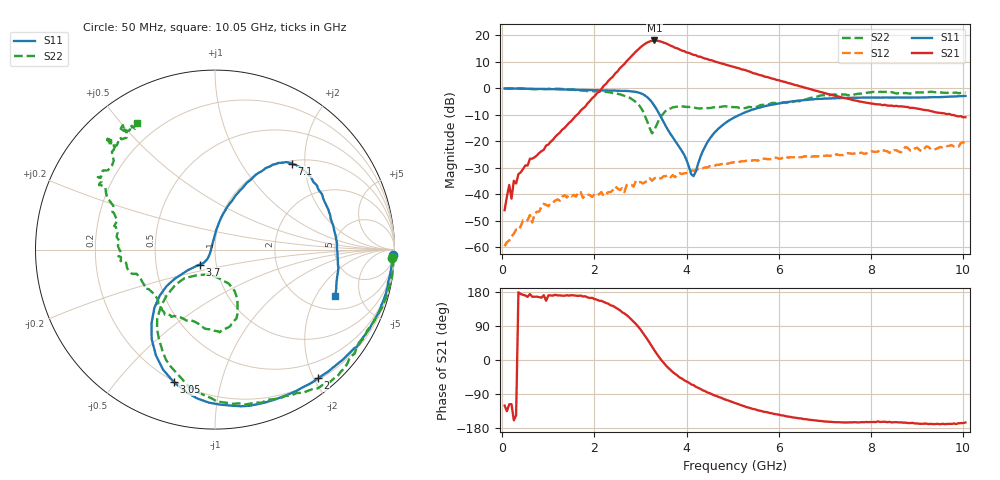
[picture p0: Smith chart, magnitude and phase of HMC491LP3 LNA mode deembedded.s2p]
!Hittite Microwave Corporation
!12 Elizabeth Drive
!Chelmsford, MA 01824
!Tel: 978-250-3343
!Fax: 978-250-3373
!Device: HMC491LP3, 3.4-3.8 GHz, GaAs MMIC Low Noise Amplifier with Bypass Mode in leadless SMT package
!Misc: LNA Mode, Room
# MHZ S MA R 50
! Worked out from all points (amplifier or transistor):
!   201 points, 50 MHz to 10.05 GHz, reference 50 ohm
!   highest |S21| = 18.0 dB at 3.3 GHz (marker M1)
!   |S21| within 3 dB of that: 2.973 GHz to 3.802 GHz (828.6 MHz wide, 24.5 % of centre)
!   unconditionally stable (mu >= 1): start of sweep to 1.123 GHz; 1.331 GHz to 2.286 GHz; 2.979 GHz to end of sweep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
!   at 1.7 GHz: K = 2.02, MAG = 9.6 dB, |S12| = -39.2 dB
!   at 5.05 GHz: K = 3.87, MAG = 9.1 dB, |S12| = -28.0 dB
!   at 10.05 GHz: K = 2.52, MAG = -1.8 dB, |S12| = -21.0 dB
!   S11 on the Smith chart (normalised r, x): 50 MHz: 17, -58; 2 GHz: 0.23, -2.06; 3.05 GHz: 0.20, -0.72; 3.7 GHz: 0.83, -0.14; 7.1 GHz: 1.06, +1.73; 10.05 GHz: 2.74, -2.93
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50  0.991 -1.8  0.005002 -120.3  0.00105 -2.1  0.99 -2.7
150  0.989 -4.2  0.015 -116.9  0.001341 61.9  0.995 -6.6
1750  0.929 -45.3  0.415 167.5  0.008565 88.3  0.904 -66.7
2000  0.918 -51.3  0.707 160.7  0.009968 73.9  0.88 -77.3
2400  0.904 -63.6  1.66 142.9  0.012 80.8  0.814 -94.1
2700  0.891 -77.5  3.256 118.4  0.015 68.5  0.695 -111.0
2900  0.853 -92.3  4.928 94.9  0.018 46.8  0.549 -126.1
3050  0.772 -107.4  6.445 71.7  0.016 22.1  0.372 -136.5
3150  0.674 -119.3  7.335 54.3  0.018 5.9  0.232 -136.8
3300  0.469 -136.1  7.988 25.8  0.02 -26.2  0.163 -81.3
3400  0.337 -143.0  7.763 8.0  0.02 -53.4  0.255 -64.7
3550  0.192 -142.9  7.056 -14.2  0.022 -76.7  0.378 -70.6
3700  0.119 -135.4  6.144 -32.0  0.023 -95.5  0.436 -78.9
3950  0.055 -131.6  5.011 -53.7  0.025 -115.7  0.452 -90.4
4150  0.022 160.0  4.272 -66.3  0.028 -127.6  0.437 -98.9
4350  0.065 94.8  3.767 -80.1  0.031 -133.7  0.423 -110.7
5050  0.287 70.8  2.496 -113.7  0.04 -148.3  0.441 -134.5
5700  0.461 62.0  1.652 -137.0  0.047 -155.6  0.497 -167.3
6750  0.62 51.5  0.928 -159.0  0.052 -151.3  0.674 153.5
7100  0.643 48.1  0.768 -163.0  0.053 -146.9  0.737 149.1
8400  0.667 30.9  0.469 -163.2  0.061 -136.2  0.834 134.3
10050  0.717 -21.2  0.284 -165.0  0.089 -127.4  0.829 121.6
